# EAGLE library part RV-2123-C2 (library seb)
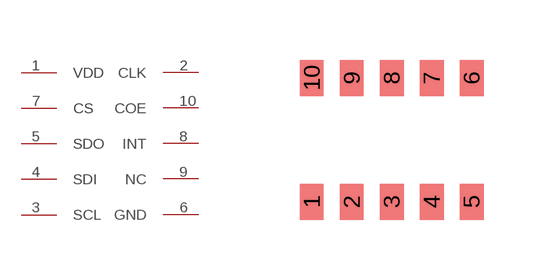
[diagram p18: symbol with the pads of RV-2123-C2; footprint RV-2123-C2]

Designator prefix IC

## RV-2123-C2  [RV-2123-C2]
1  VDD
2  CLK
3  SCL
4  SDI
5  SDO
6  GND
7  CS
8  INT
9  NC
10  COE

## Footprint RV-2123-C2 (pad centres in mm)
smd 0.6 x 0.9: 1 -2,-1.55; 2 -1,-1.55; 3 0,-1.55; 4 1,-1.55; 5 2,-1.55; 6 2,1.55; 7 1,1.55; 8 0,1.55; 9 -1,1.55; 10 -2,1.55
